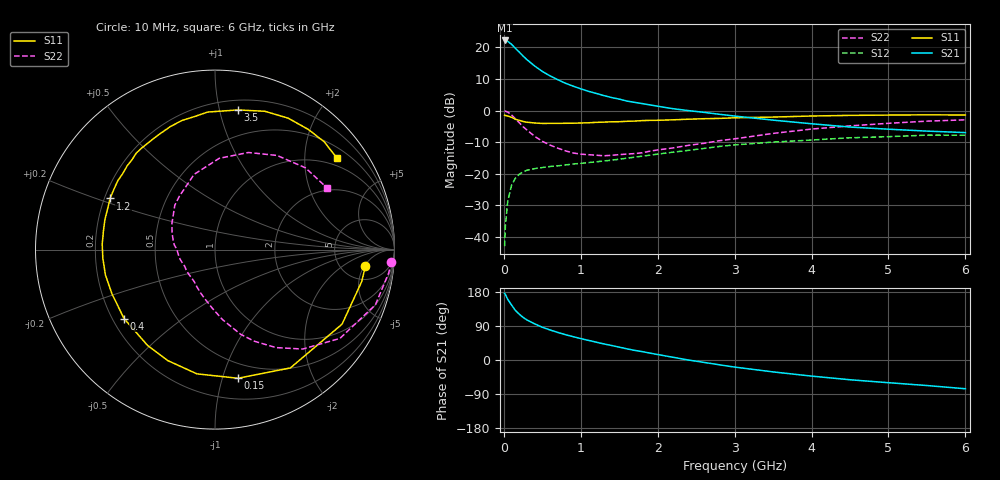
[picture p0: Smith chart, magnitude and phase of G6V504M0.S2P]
! SIEMENS Small Signal Semiconductors
! BFG193
! Si NPN RF Bipolar Junction Transistor in SOT223
! VCE = 0.5 V  IC = 4 mA
! Common Emitter S-Parameters:  August  1996
# GHz  S  MA  R  50
!  f  S11  S21  S12  S22
! GHz  MAG  ANG  MAG  ANG  MAG  ANG  MAG  ANG
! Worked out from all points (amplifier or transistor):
!   36 points, 10 MHz to 6 GHz, reference 50 ohm
!   highest |S21| = 22.1 dB at 10 MHz (marker M1)
!   |S21| within 3 dB of that: start of sweep to 171.6 MHz
!   unconditionally stable (mu >= 1): 1.085 GHz to end of sweep
!   at 250 MHz: K = 0.31, MSG = 18.3 dB, |S12| = -19.4 dB
!   at 1.4 GHz: K = 1.11, MAG = 7.8 dB, |S12| = -15.7 dB
!   at 6 GHz: K = 1.02, MAG = -0.5 dB, |S12| = -7.8 dB
!   S11 on the Smith chart (normalised r, x): 10 MHz: 8.31, -5.33; 150 MHz: 0.37, -1.12; 400 MHz: 0.25, -0.32; 1.2 GHz: 0.22, +0.22; 3.5 GHz: 0.28, +1.14; 6 GHz: 0.77, +2.82
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0.01  0.8433 -6.3  12.79 175.9  0.0072 89.7  0.9855 -3.9
0.02  0.8363 -12.4  12.76 173.0  0.0149 84.5  0.9764 -7.7
0.05  0.8208 -30.4  12.38 160.3  0.0365 73.5  0.9451 -19.0
0.1  0.7817 -57.5  11.13 145.2  0.0659 61.0  0.8541 -35.4
0.15  0.7281 -79.9  9.604 130.8  0.0854 50.2  0.7386 -48.6
0.2  0.6995 -98.3  8.379 121.0  0.0984 43.2  0.6431 -58.1
0.25  0.672 -113.0  7.249 112.4  0.1074 37.6  0.5543 -66.9
0.3  0.6532 -125.0  6.362 105.7  0.1137 33.9  0.4925 -73.2
0.4  0.6358 -142.8  5.06 95.4  0.1209 29.0  0.392 -83.9
0.5  0.6248 -156.7  4.147 86.5  0.1258 25.8  0.3266 -92.7
0.6  0.6265 -166.9  3.531 79.3  0.1305 24.3  0.2848 -100.5
0.7  0.6269 -175.6  3.072 72.8  0.1337 23.3  0.2548 -108.3
0.9  0.6301 170.6  2.43 61.6  0.1429 22.4  0.2136 -122.5
1.1  0.6399 159.3  2.013 51.8  0.1504 22.2  0.2006 -137.1
1.2  0.6503 154.0  1.864 47.1  0.1547 22.1  0.1968 -144.2
1.6  0.6761 136.4  1.412 29.5  0.1767 20.9  0.2051 -170.1
2.2  0.7133 116.0  1.069 7.2  0.2198 15.7  0.2567 158.7
2.8  0.7509 98.3  0.873 -12.6  0.2706 6.8  0.3335 132.2
3.5  0.7884 80.7  0.705 -31.4  0.3173 -8.1  0.4351 105.5
4.5  0.8381 60.9  0.548 -52.1  0.371 -26.6  0.5722 71.0
5.5  0.8551 44.6  0.473 -67.4  0.4086 -49.1  0.6795 42.1
6  0.8495 36.7  0.448 -75.9  0.4076 -61.9  0.7128 28.8
